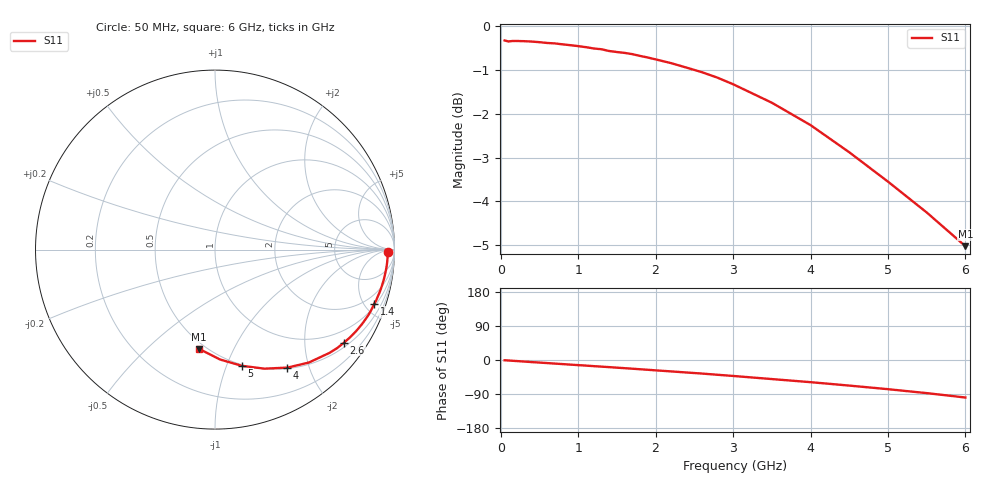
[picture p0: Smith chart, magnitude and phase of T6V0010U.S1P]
! SIEMENS Discrete & RF Semiconductors
! BAT62
! Si Schottky Diode in SOT143
! IF = 0.01 mA
! S-Parameters:  February  1997
# GHz  S  MA  R  50
!  f  S11
! GHz  MAG  ANG
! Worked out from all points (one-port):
!   34 points, 50 MHz to 6 GHz, reference 50 ohm
!   lowest |S11| = -5.0 dB at 6 GHz (marker M1), VSWR 3.55, Z = 23 - j37.2 ohm
!   |S11| at or under -10 dB: nowhere
!   S11 on the Smith chart (normalised r, x): 50 MHz: 49, -16; 1.4 GHz: 1.17, -5.81; 2.6 GHz: 0.62, -2.98; 4 GHz: 0.51, -1.67; 5 GHz: 0.49, -1.13; 6 GHz: 0.46, -0.74
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0.05  0.9637 -0.7
0.1  0.9612 -1.3
0.15  0.9624 -2.0
0.2  0.9624 -2.7
0.4  0.9609 -5.5
0.6  0.9573 -8.1
0.7  0.9562 -9.5
0.8  0.9539 -10.8
0.9  0.9517 -12.2
1.1  0.9468 -14.8
1.2  0.9436 -16.2
1.3  0.9417 -17.5
1.4  0.9373 -18.8
1.6  0.9326 -21.6
1.7  0.9296 -23.0
1.9  0.9213 -25.8
2  0.9169 -27.3
2.2  0.9078 -30.1
2.4  0.8971 -33.0
2.6  0.8863 -35.8
2.8  0.8737 -39.0
3  0.8588 -42.1
3.5  0.818 -50.3
4  0.7712 -58.5
4.5  0.718 -67.5
5  0.6646 -77.0
5.5  0.6128 -87.4
6  0.5607 -99.0
